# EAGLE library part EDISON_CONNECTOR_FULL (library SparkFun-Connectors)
Intel &reg; Edison Hirose Connectors DF40 Series 70 pin connector 3mm headers and sockets used on the SparkFun Edison Blocks. Edison Daughter package includes layout for the Edison module itself, including mounting holes and antenna area marked. SparkFun Products: SparkFun ADC Edison Block SparkFun Power Edison Block SparkFun Base Edison Block SparkFun Dual H-Bridge Edison Block SparkFun microSD Edison Block
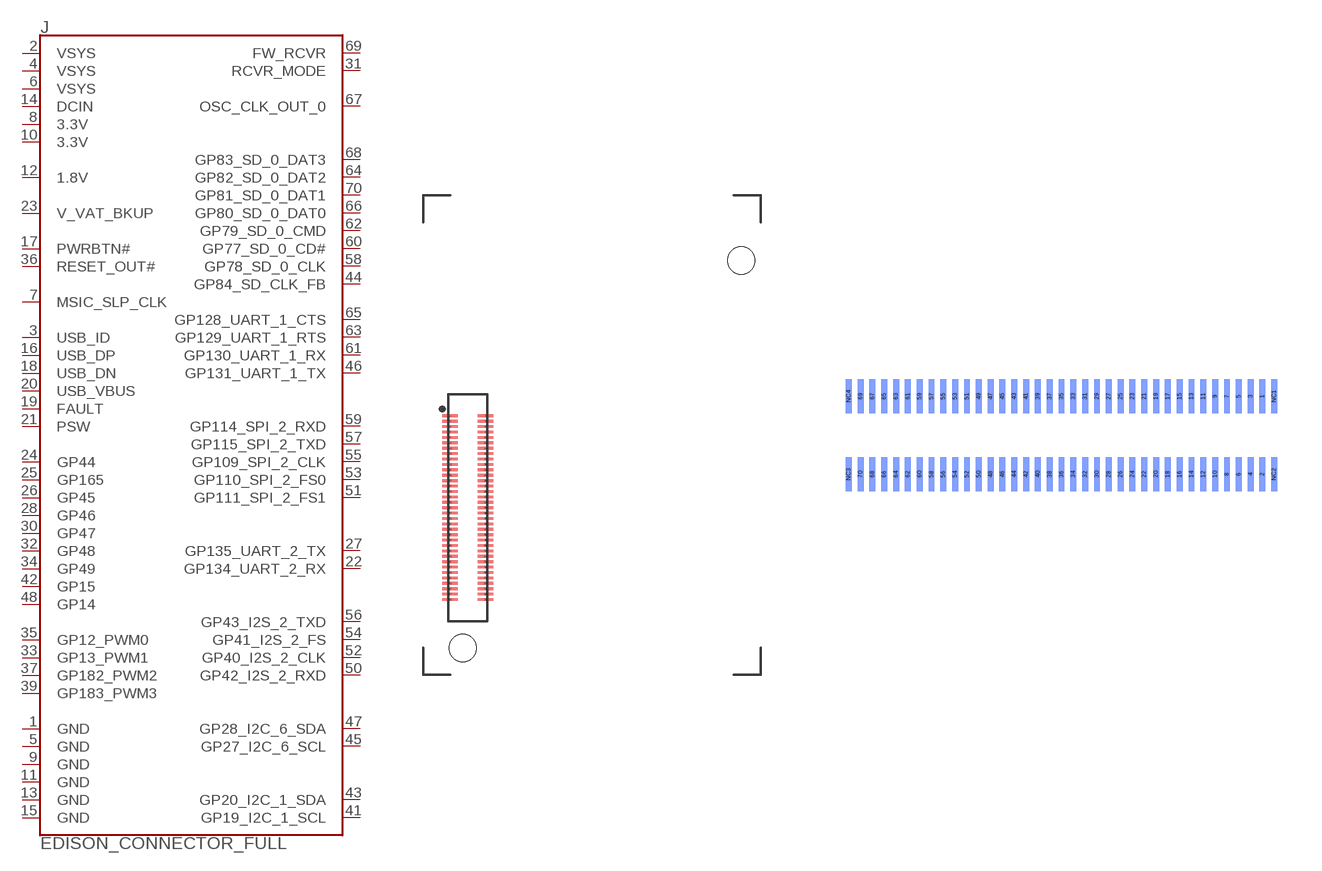
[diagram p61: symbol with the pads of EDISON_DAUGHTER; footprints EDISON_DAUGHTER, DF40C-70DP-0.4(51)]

Designator prefix J

## EDISON_CONNECTOR_FULL_MOUNTING_HOLES  [EDISON_DAUGHTER]
1  GND
2  VSYS
3  USB_ID
4  VSYS
5  GND
6  VSYS
7  MSIC_SLP_CLK
8  3.3V
9  GND
10  3.3V
11  GND
12  1.8V
13  GND
14  DCIN
15  GND
16  USB_DP
17  PWRBTN#
18  USB_DN
19  FAULT
20  USB_VBUS
21  PSW
22  GP134_UART_2_RX
23  V_VAT_BKUP
24  GP44
25  GP165
26  GP45
27  GP135_UART_2_TX
28  GP46
30  GP47
31  RCVR_MODE
32  GP48
33  GP13_PWM1
34  GP49
35  GP12_PWM0
36  RESET_OUT#
37  GP182_PWM2
39  GP183_PWM3
41  GP19_I2C_1_SCL
42  GP15
43  GP20_I2C_1_SDA
44  GP84_SD_CLK_FB
45  GP27_I2C_6_SCL
46  GP131_UART_1_TX
47  GP28_I2C_6_SDA
48  GP14
50  GP42_I2S_2_RXD
51  GP111_SPI_2_FS1
52  GP40_I2S_2_CLK
53  GP110_SPI_2_FS0
54  GP41_I2S_2_FS
55  GP109_SPI_2_CLK
56  GP43_I2S_2_TXD
57  GP115_SPI_2_TXD
58  GP78_SD_0_CLK
59  GP114_SPI_2_RXD
60  GP77_SD_0_CD#
61  GP130_UART_1_RX
62  GP79_SD_0_CMD
63  GP129_UART_1_RTS
64  GP82_SD_0_DAT2
65  GP128_UART_1_CTS
66  GP80_SD_0_DAT0
67  OSC_CLK_OUT_0
68  GP83_SD_0_DAT3
69  FW_RCVR
70  GP81_SD_0_DAT1

## EDISON_CONNECTOR_FULL_HEADER (PROD_ID: CONN-12248)  [DF40C-70DP-0.4(51)]
Pads as for EDISON_DAUGHTER

## EDISON_CONNECTOR_FULL_SOCKET (PROD_ID: CONN-12247)  [DF40-XC-(X.X)-70DS-0.4V(51)]
Pads as for EDISON_DAUGHTER

## Footprint EDISON_DAUGHTER (pad centres in mm)
Hirose DF30C-70DP-0.4V(51) Receiver Footprint w/ Edison Outline Package can be used as basic guideline for creating Edison-mating daughter boards. Includes keepout area for antenna. Specifications: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
smd 1.14 x 0.2: 1 1.98,19.17; 2 4.62,19.17; 3 1.98,18.77; 4 4.62,18.77; 5 1.98,18.37; 6 4.62,18.37; 7 1.98,17.97; 8 4.62,17.97; 9 1.98,17.57; 10 4.62,17.57; 11 1.98,17.17; 12 4.62,17.17; 13 1.98,16.77; 14 4.62,16.77; 15 1.98,16.37; 16 4.62,16.37; 17 1.98,15.97; 18 4.62,15.97; 19 1.98,15.57; 20 4.62,15.57; 21 1.98,15.17; 22 4.62,15.17; 23 1.98,14.77; 24 4.62,14.77; 25 1.98,14.37; 26 4.62,14.37; 27 1.98,13.97; 28 4.62,13.97; 29 1.98,13.57; 30 4.62,13.57; 31 1.98,13.17; 32 4.62,13.17; 33 1.98,12.77; 34 4.62,12.77; 35 1.98,12.37; 36 4.62,12.37; 37 1.98,11.97; 38 4.62,11.97; 39 1.98,11.57; 40 4.62,11.57; 41 1.98,11.17; 42 4.62,11.17; 43 1.98,10.77; 44 4.62,10.77; 45 1.98,10.37; 46 4.62,10.37; 47 1.98,9.97; 48 4.62,9.97; 49 1.98,9.57; 50 4.62,9.57; 51 1.98,9.17; 52 4.62,9.17; 53 1.98,8.77; 54 4.62,8.77; 55 1.98,8.37; 56 4.62,8.37; 57 1.98,7.97; 58 4.62,7.97; 59 1.98,7.57; 60 4.62,7.57; 61 1.98,7.17; 62 4.62,7.17; 63 1.98,6.77; 64 4.62,6.77; 65 1.98,6.37; 66 4.62,6.37; 67 1.98,5.97; 68 4.62,5.97; 69 1.98,5.57; 70 4.62,5.57
hole 2 at 23.53,30.67
hole 2 at 2.93,1.98

## Footprint DF40C-70DP-0.4(51) (pad centres in mm)
Hirose DF30C-70DP-0.4V(51) Receiver Specifications: Pin count:70 Pin pitch: 0.4mm Datasheet referenced for footprint Example device(s): EDISON_FULL_CONNECTOR
smd 0.2 x 1.14 bottom: 1 6.8,1.32; 2 6.8,-1.32; 3 6.4,1.32; 4 6.4,-1.32; 5 6,1.32; 6 6,-1.32; 7 5.6,1.32; 8 5.6,-1.32; 9 5.2,1.32; 10 5.2,-1.32; 11 4.8,1.32; 12 4.8,-1.32; 13 4.4,1.32; 14 4.4,-1.32; 15 4,1.32; 16 4,-1.32; 17 3.6,1.32; 18 3.6,-1.32; 19 3.2,1.32; 20 3.2,-1.32; 21 2.8,1.32; 22 2.8,-1.32; 23 2.4,1.32; 24 2.4,-1.32; 25 2,1.32; 26 2,-1.32; 27 1.6,1.32; 28 1.6,-1.32; 29 1.2,1.32; 30 1.2,-1.32; 31 0.8,1.32; 32 0.8,-1.32; 33 0.4,1.32; 34 0.4,-1.32; 35 0,1.32; 36 0,-1.32; 37 -0.4,1.32; 38 -0.4,-1.32; 39 -0.8,1.32; 40 -0.8,-1.32; 41 -1.2,1.32; 42 -1.2,-1.32; 43 -1.6,1.32; 44 -1.6,-1.32; 45 -2,1.32; 46 -2,-1.32; 47 -2.4,1.32; 48 -2.4,-1.32; 49 -2.8,1.32; 50 -2.8,-1.32; 51 -3.2,1.32; 52 -3.2,-1.32; 53 -3.6,1.32; 54 -3.6,-1.32; 55 -4,1.32; 56 -4,-1.32; 57 -4.4,1.32; 58 -4.4,-1.32; 59 -4.8,1.32; 60 -4.8,-1.32; 61 -5.2,1.32; 62 -5.2,-1.32; 63 -5.6,1.32; 64 -5.6,-1.32; 65 -6,1.32; 66 -6,-1.32; 67 -6.4,1.32; 68 -6.4,-1.32; 69 -6.8,1.32; 70 -6.8,-1.32; NC1 7.2,1.32; NC2 7.2,-1.32; NC3 -7.2,-1.32; NC4 -7.2,1.32

## Footprint DF40-XC-(X.X)-70DS-0.4V(51) (pad centres in mm)
Hirose DF40C-70DP-0.4V(51) Plug Specifications: Pin count:70 Pin pitch: 0.4mm Datasheet referenced for footprint Example device(s): EDISON_FULL_CONNECTOR
smd 0.2 x 1.14: 1 6.8,1.32; 2 6.8,-1.32; 3 6.4,1.32; 4 6.4,-1.32; 5 6,1.32; 6 6,-1.32; 7 5.6,1.32; 8 5.6,-1.32; 9 5.2,1.32; 10 5.2,-1.32; 11 4.8,1.32; 12 4.8,-1.32; 13 4.4,1.32; 14 4.4,-1.32; 15 4,1.32; 16 4,-1.32; 17 3.6,1.32; 18 3.6,-1.32; 19 3.2,1.32; 20 3.2,-1.32; 21 2.8,1.32; 22 2.8,-1.32; 23 2.4,1.32; 24 2.4,-1.32; 25 2,1.32; 26 2,-1.32; 27 1.6,1.32; 28 1.6,-1.32; 29 1.2,1.32; 30 1.2,-1.32; 31 0.8,1.32; 32 0.8,-1.32; 33 0.4,1.32; 34 0.4,-1.32; 35 0,1.32; 36 0,-1.32; 37 -0.4,1.32; 38 -0.4,-1.32; 39 -0.8,1.32; 40 -0.8,-1.32; 41 -1.2,1.32; 42 -1.2,-1.32; 43 -1.6,1.32; 44 -1.6,-1.32; 45 -2,1.32; 46 -2,-1.32; 47 -2.4,1.32; 48 -2.4,-1.32; 49 -2.8,1.32; 50 -2.8,-1.32; 51 -3.2,1.32; 52 -3.2,-1.32; 53 -3.6,1.32; 54 -3.6,-1.32; 55 -4,1.32; 56 -4,-1.32; 57 -4.4,1.32; 58 -4.4,-1.32; 59 -4.8,1.32; 60 -4.8,-1.32; 61 -5.2,1.32; 62 -5.2,-1.32; 63 -5.6,1.32; 64 -5.6,-1.32; 65 -6,1.32; 66 -6,-1.32; 67 -6.4,1.32; 68 -6.4,-1.32; 69 -6.8,1.32; 70 -6.8,-1.32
